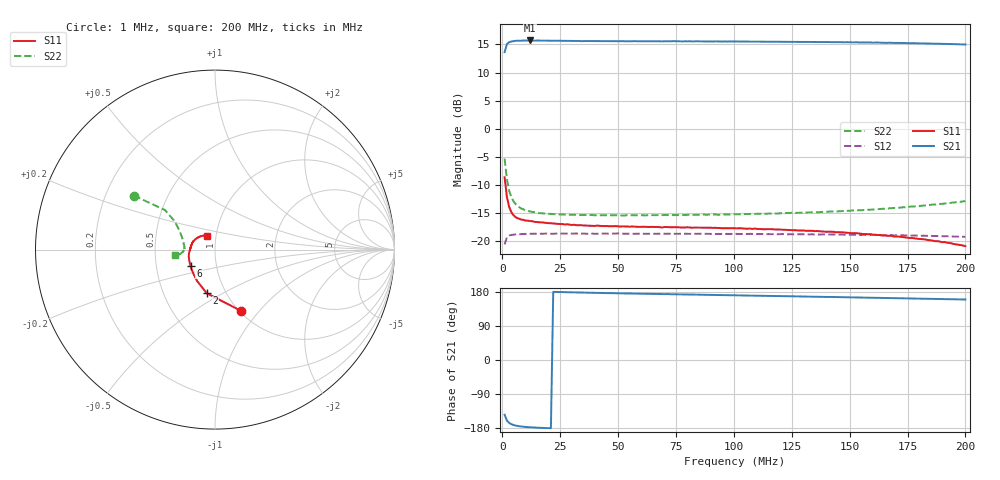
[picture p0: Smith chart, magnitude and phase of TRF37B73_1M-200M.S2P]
!Agilent Technologies,E5071B,JP1KK00322,A.09.10
!Date: Wed Jul 02 14:17:08 2014
!Data & Calibration Information:
!Freq		S11:SOLT2(ON)  S21:SOLT2(ON)  S12:SOLT2(ON)  S22:SOLT2(ON)
# Hz S dB R 50
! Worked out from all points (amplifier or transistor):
!   200 points, 1 MHz to 200 MHz, reference 50 ohm
!   highest |S21| = 15.7 dB at 12 MHz (marker M1)
!   |S21| within 3 dB of that: start of sweep to end of sweep
!   unconditionally stable (mu >= 1): start of sweep to end of sweep
!   at 34 MHz: K = 1.05, MAG = 15.7 dB, |S12| = -18.6 dB
!   at 101 MHz: K = 1.05, MAG = 15.6 dB, |S12| = -18.6 dB
!   at 200 MHz: K = 1.09, MAG = 15.2 dB, |S12| = -19.2 dB
!   S11 on the Smith chart (normalised r, x): 1 MHz: 1.02, -0.81; 2 MHz: 0.81, -0.42; 6 MHz: 0.75, -0.14; 200 MHz: 0.90, +0.14
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1000000  -8.61 -67.0  13.63 -144.3  -20.53 38.7  -5.28 146.4
2000000  -12.13 -100.7  15.06 -159.8  -19.25 21.4  -8.98 141.7
3000000  -13.92 -119.7  15.40 -166.2  -18.95 14.7  -11.05 144.6
4000000  -14.88 -132.0  15.52 -169.7  -18.83 11.0  -12.22 148.5
5000000  -15.41 -140.6  15.59 -171.8  -18.78 8.9  -12.97 151.9
6000000  -15.77 -146.7  15.64 -173.4  -18.74 7.4  -13.48 154.9
8000000  -16.10 -155.1  15.65 -175.3  -18.69 5.3  -14.11 159.2
1.2e7  -16.39 -164.0  15.70 -177.5  -18.64 3.2  -14.68 164.6
1.9e7  -16.72 -172.0  15.66 -179.7  -18.59 1.4  -15.02 170.0
3.5e7  -17.16 179.7  15.59 177.8  -18.59 -1.0  -15.29 174.9
6.8e7  -17.47 169.9  15.54 174.1  -18.64 -4.0  -15.33 179.2
7e7  -17.44 169.2  15.55 173.7  -18.63 -4.3  -15.32 179.2
7.2e7  -17.46 168.9  15.55 173.9  -18.62 -4.2  -15.31 179.5
7.3e7  -17.48 168.4  15.56 173.3  -18.63 -4.7  -15.32 179.4
8.2e7  -17.56 166.1  15.52 172.7  -18.63 -5.3  -15.28 -179.7
1.01e8  -17.68 161.6  15.52 170.6  -18.65 -6.8  -15.18 -178.1
1.34e8  -18.11 152.5  15.43 167.0  -18.73 -9.3  -14.82 -175.6
1.41e8  -18.26 150.5  15.42 166.5  -18.77 -10.1  -14.70 -175.1
1.67e8  -19.00 140.8  15.30 163.5  -18.87 -12.4  -14.12 -172.9
1.78e8  -19.45 135.0  15.21 162.0  -18.95 -13.4  -13.77 -172.0
1.79e8  -19.51 134.6  15.20 162.2  -18.96 -13.5  -13.73 -171.8
2e8  -20.84 120.8  14.98 159.6  -19.17 -15.4  -12.85 -171.9
